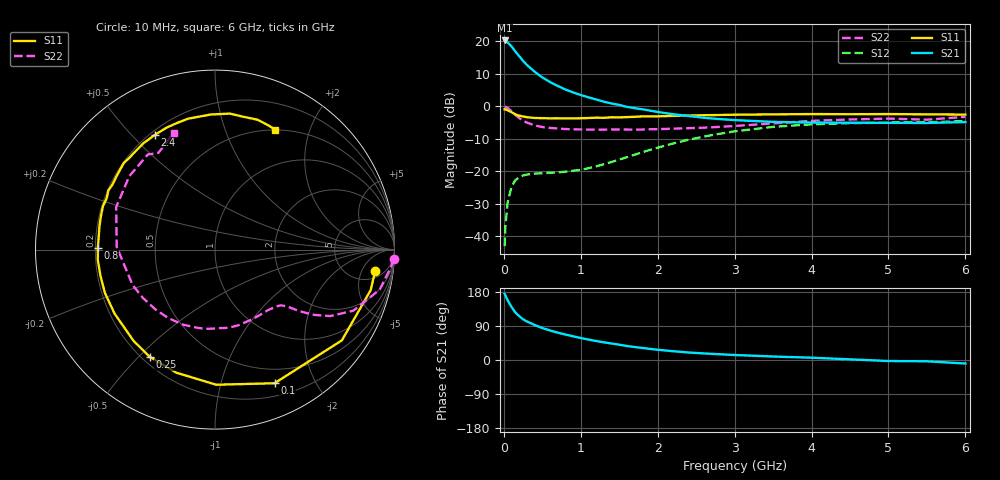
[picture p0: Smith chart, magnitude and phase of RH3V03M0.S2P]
! SIEMENS Small Signal Semiconductors
! BFR106
! Si NPN RF Bipolar Junction Transistor in SOT23
! VCE = 3 V  IC = 3 mA
! Common Emitter S-Parameters:  August  1996
# GHz  S  MA  R  50
!  f  S11  S21  S12  S22
! GHz  MAG  ANG  MAG  ANG  MAG  ANG  MAG  ANG
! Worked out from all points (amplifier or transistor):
!   36 points, 10 MHz to 6 GHz, reference 50 ohm
!   highest |S21| = 20.3 dB at 10 MHz (marker M1)
!   |S21| within 3 dB of that: start of sweep to 136.9 MHz
!   unconditionally stable (mu >= 1): 719.9 MHz to 2.045 GHz; 4.067 GHz to end of sweep
!   at 250 MHz: K = 0.39, MSG = 17.6 dB, |S12| = -21.2 dB
!   at 1.4 GHz: K = 1.20, MAG = 6.3 dB, |S12| = -17.1 dB
!   at 6 GHz: K = 1.02, MAG = -1.1 dB, |S12| = -4.5 dB
!   S11 on the Smith chart (normalised r, x): 10 MHz: 7, -9; 100 MHz: 0.34, -1.49; 250 MHz: 0.23, -0.54; 800 MHz: 0.21, +0.01; 2.4 GHz: 0.22, +0.59; 6 GHz: 0.50, +1.51
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0.01  0.9006 -7.5  10.31 174.7  0.0071 88.0  0.9961 -3.0
0.02  0.8963 -14.6  10.16 170.9  0.0143 83.8  0.9854 -5.7
0.05  0.8691 -35.6  9.599 157.3  0.0336 71.5  0.9445 -13.6
0.1  0.8151 -66.0  8.353 139.9  0.0584 56.8  0.8429 -23.8
0.15  0.7529 -89.5  6.956 125.3  0.0734 46.0  0.7409 -30.0
0.2  0.7189 -107.5  5.909 115.7  0.0816 39.7  0.6627 -33.3
0.25  0.6992 -121.4  5.011 107.5  0.0868 35.3  0.601 -35.4
0.3  0.6816 -131.7  4.331 101.7  0.0894 33.0  0.5634 -36.6
0.4  0.6635 -147.5  3.412 92.3  0.0926 30.4  0.51 -38.3
0.5  0.6593 -158.5  2.789 84.4  0.0938 30.4  0.4809 -40.2
0.6  0.6546 -167.3  2.368 77.9  0.0955 31.9  0.4664 -42.7
0.8  0.6528 179.1  1.819 67.2  0.099 37.4  0.4486 -48.7
1.1  0.6627 163.4  1.376 53.9  0.112 49.0  0.4397 -60.1
1.3  0.6678 154.7  1.181 46.6  0.1293 55.7  0.4388 -68.4
1.6  0.6843 143.3  0.982 36.9  0.1656 61.7  0.4408 -82.1
2.2  0.7144 123.8  0.757 23.2  0.2688 60.8  0.4543 -112.8
2.4  0.7219 117.5  0.712 19.8  0.3068 58.0  0.462 -124.4
3.5  0.753 91.8  0.578 9.2  0.4841 35.5  0.5479 178.4
4.5  0.7567 77.5  0.561 1.7  0.5515 15.1  0.6287 139.4
5  0.7615 72.0  0.558 -2.7  0.5636 7.3  0.6487 125.2
5.5  0.7534 66.8  0.556 -3.4  0.5698 3.5  0.6246 120.3
6  0.7479 63.3  0.574 -9.3  0.5937 -4.3  0.6908 109.3
